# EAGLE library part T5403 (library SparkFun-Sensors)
Epcos T5403 Digital Barometric Pressure Sensor The T5403 sensor measures the absolute pressure of the air around. This pressure varies with both the weather and altitude. Depending on how you interpret the data, you can monitor changes in the weather, measure altitude, or any other tasks that require an accurate pressure reading. Datasheet SparkFun Products SparkFun Barometric Sensor Breakout - T5403 (SEN-12039)
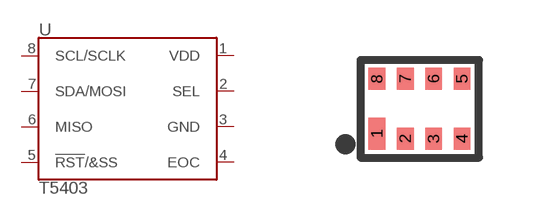
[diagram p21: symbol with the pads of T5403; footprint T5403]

Designator prefix U

## T5403 (PROD_ID: IC-11772)  [T5403]
1  VDD
2  SEL
3  GND
4  EOC
5  !RST!/&SS
6  MISO
7  SDA/MOSI
8  SCL/SCLK

## Footprint T5403 (pad centres in mm)
T5400, T54003 Digital Barometric Pressure Sensor Datasheet Specifications: Pin Count: 8 Area: 2.78 x 2.23 x 0.5 mm Pitch: 0.71 mm Devices Using: T5403
smd 0.42 x 0.8: 1 -1.065,-0.625
smd 0.42 x 0.55: 2 -0.355,-0.75; 3 0.355,-0.75; 4 1.065,-0.75; 5 1.065,0.75; 6 0.355,0.75; 7 -0.355,0.75; 8 -1.065,0.75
